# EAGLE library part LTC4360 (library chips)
An overvoltage protection IC. Clamps at 5.5V
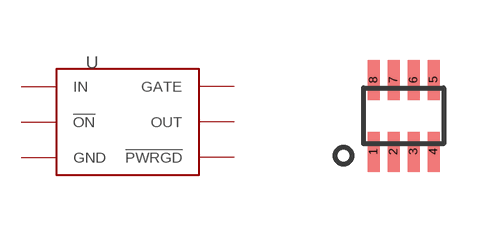
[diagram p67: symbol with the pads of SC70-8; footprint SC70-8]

Designator prefix U

## LTC4360 (DIGIKEY: LTC4360CSC8-1#TRMPBFCT-ND)  [SC70-8]
1  IN
2  GND
3  GND
4  GND
5  !PWRGD
6  !ON
7  OUT
8  GATE

## Footprint SC70-8 (pad centres in mm)
smd 0.3 x 1: 1 -0.75,-0.9; 2 -0.25,-0.9; 3 0.25,-0.9; 4 0.75,-0.9; 5 0.75,0.9; 6 0.25,0.9; 7 -0.25,0.9; 8 -0.75,0.9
